(* Logix 5000 AddOnInstructionDefinition export SPEL_Pallet4Get; software revision 30.01 *)

ADD_ON_INSTRUCTION SPEL_ExecCmd   (* revision 1.0 *)
// Executes a command in the robot controller.  Normally this is called by higher level AOIs.
VAR_INPUT
   Start : BOOL; {required}
   MaxTime : DINT := 3000; {required}
END_VAR
VAR_OUTPUT
   InCycle : BOOL; {access Read Only, visible}
   Done : BOOL; {access Read Only, visible}
   Error : BOOL; {access Read Only, visible}
END_VAR
VAR_IN_OUT
   ExtInputs : AB:ETHERNET_MODULE_INT_128Bytes:I:0; {required}
        .DATA[0].0   // ExtCmdGet
        .DATA[0].1   // ExtRespSet
        .DATA[0].2   // ExtCmdResult
        .DATA[0].3   // ExtError
   ExtOutputs : AB:ETHERNET_MODULE_INT_128Bytes:O:0; {required}
        .DATA[0].0   // ExtCmdSet
        .DATA[0].1   // ExtRespGet
        .DATA[0].2   // ExtCmdReset
END_VAR
VAR_INPUT
   Cmd : INT; {required}
   CmdParam1 : INT; {required}
   CmdParam2 : INT; {required}
   CmdParam3 : INT; {required}
   CmdParam4 : INT; {required}
   CmdParam5 : INT; {required}
   CmdParam6 : INT; {required}
   CmdParam7 : INT; {required}
END_VAR
VAR_OUTPUT
   CmdEcho : INT; {access Read Only, visible}
   Resp1 : INT; {access Read Only, visible}
   Resp2 : INT; {access Read Only, visible}
   Resp3 : INT; {access Read Only, visible}
   Resp4 : INT; {access Read Only, visible}
   Resp5 : INT; {access Read Only, visible}
   Resp6 : INT; {access Read Only, visible}
   Resp7 : INT; {access Read Only, visible}
   ErrCode1 : INT; {access Read Only, visible}
   ErrCode2 : INT; {access Read Only, visible}
END_VAR
VAR
   ExtReset : BOOL; {access None}
   ExtError : BOOL; {access None}
   ExtCmdSet : BOOL; {access None}   // Cmd Ready
   ExtCmdGet : BOOL; {access None}   // Cmd Received
   CmdXferDone : BOOL; {access None}
   ExtRespSet : BOOL; {access None}   // Resp Ready
   RespXferDone : BOOL; {access None}
   ExtCmdResult : BOOL; {access None}   // Normal or Error?
   TmrCmdDataRdy : TIMER := (PRE := 5); {access None}
   OneShotDoneOff : BOOL; {access None}
   OneShotStart : BOOL; {access None}
   StartInit : BOOL; {access None}
   OneShotStartError : BOOL; {access None}
   TmrCycle : TIMER := (PRE := 5000); {access None}
   OneshotTmrPreset : BOOL; {access None}
   TmrCmdSet : TIMER := (PRE := 20); {access None}
   OnShotCmdDataXfer : BOOL; {access None}
   OneShotRespDataXfer : BOOL; {access None}
   OneShotDataRdy : BOOL; {access None}
   OtherCmdInCycle : BOOL; {access None}
   s : BOOL; {access None}
   OneShotUnsetCmdIncycle : BOOL; {access None}
   OneShotSetCmdIncycle : BOOL; {access None}
   OneShotSetOtherCmdInCycleError : BOOL; {access None}
   OneShotSetBit : BOOL; {access None}
   MaxTimeError : BOOL; {access None}
END_VAR

ROUTINE Logic   (* ladder *)
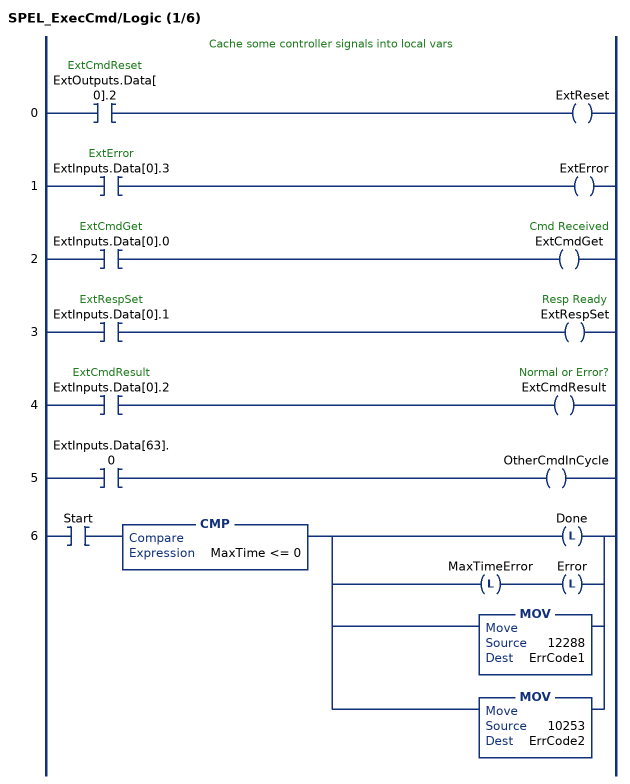
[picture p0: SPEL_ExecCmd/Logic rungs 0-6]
   // Cache some controller signals into local vars
   0: XIC(ExtOutputs.Data[0].2)OTE(ExtReset);
   1: XIC(ExtInputs.Data[0].3)OTE(ExtError);
   2: XIC(ExtInputs.Data[0].0)OTE(ExtCmdGet);
   3: XIC(ExtInputs.Data[0].1)OTE(ExtRespSet);
   4: XIC(ExtInputs.Data[0].2)OTE(ExtCmdResult);
   5: XIC(ExtInputs.Data[63].0)OTE(OtherCmdInCycle);
   6: XIC(Start)CMP(MaxTime <= 0)[OTL(Done) ,OTL(MaxTimeError) OTL(Error) ,MOV(12288,ErrCode1) ,MOV(10253,ErrCode2) ];
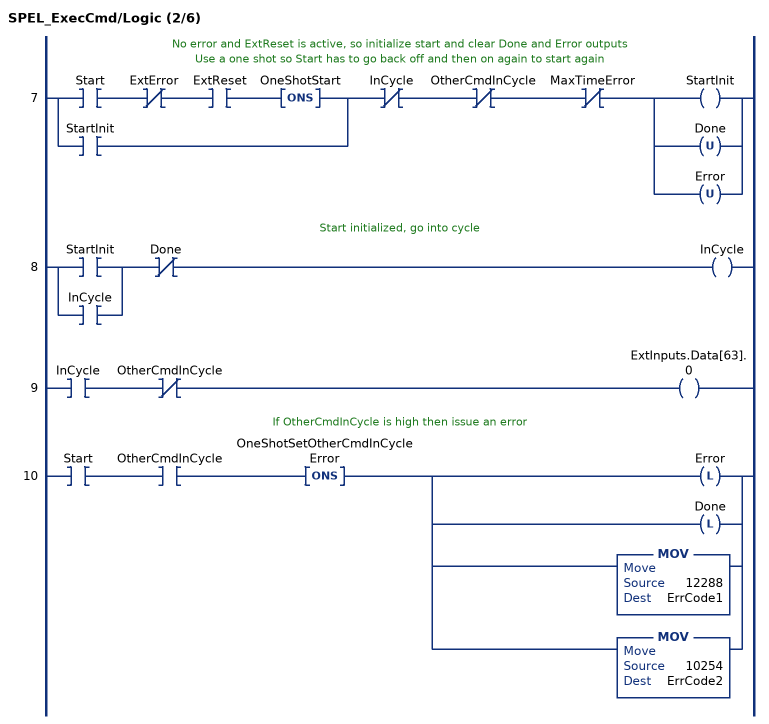
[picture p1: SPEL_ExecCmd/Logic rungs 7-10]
   // No error and ExtReset is active, so initialize start and clear Done and Error outputs
   // Use a one shot so Start has to go back off and then on again to start again
   7: [XIC(Start) XIO(ExtError) XIC(ExtReset) ONS(OneShotStart) ,XIC(StartInit) ]XIO(InCycle)XIO(OtherCmdInCycle)XIO(MaxTimeError)[OTE(StartInit) ,OTU(Done) ,OTU(Error) ];
   // Start initialized, go into cycle
   8: [XIC(StartInit) ,XIC(InCycle) ]XIO(Done)OTE(InCycle);
   9: XIC(InCycle)XIO(OtherCmdInCycle)OTE(ExtInputs.Data[63].0);
   // If OtherCmdInCycle is high then issue an error
   10: XIC(Start)XIC(OtherCmdInCycle)ONS(OneShotSetOtherCmdInCycleError)[OTL(Error) ,OTL(Done) ,MOV(12288,ErrCode1) ,MOV(10254,ErrCode2) ];
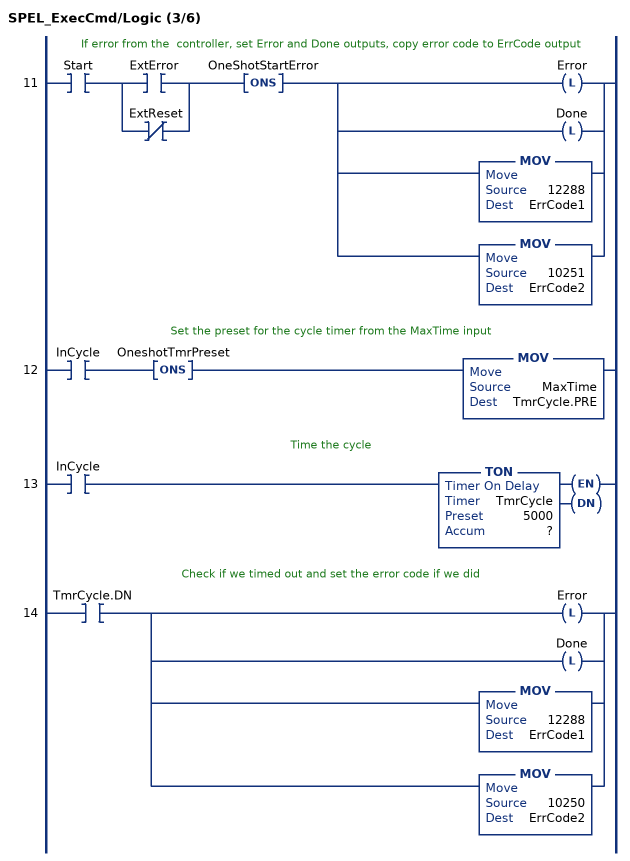
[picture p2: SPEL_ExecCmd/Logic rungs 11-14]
   // If error from the  controller, set Error and Done outputs, copy error code to ErrCode output
   11: XIC(Start)[XIC(ExtError) ,XIO(ExtReset) ]ONS(OneShotStartError)[OTL(Error) ,OTL(Done) ,MOV(12288,ErrCode1) ,MOV(10251,ErrCode2) ];
   // Set the preset for the cycle timer from the MaxTime input
   12: XIC(InCycle)ONS(OneshotTmrPreset)MOV(MaxTime,TmrCycle.PRE);
   // Time the cycle
   13: XIC(InCycle)TON(TmrCycle,?,?);
   // Check if we timed out and set the error code if we did
   14: XIC(TmrCycle.DN)[OTL(Error) ,OTL(Done) ,MOV(12288,ErrCode1) ,MOV(10250,ErrCode2) ];
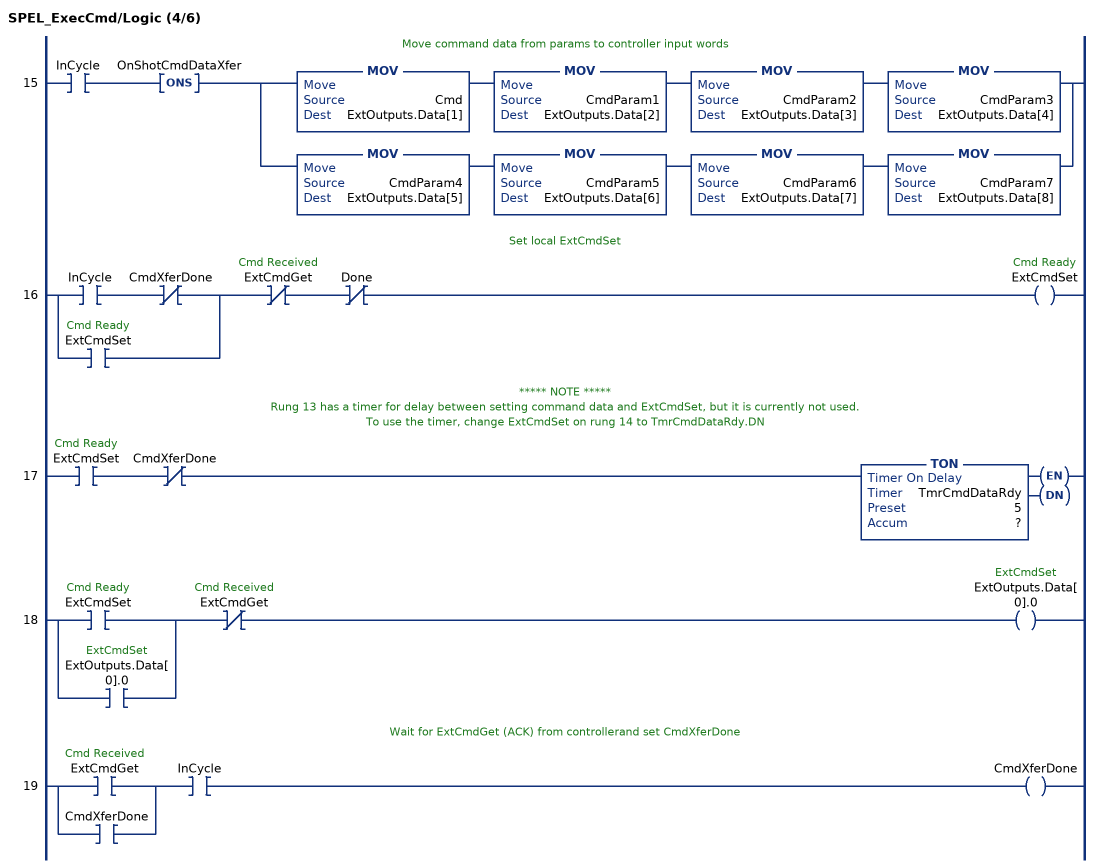
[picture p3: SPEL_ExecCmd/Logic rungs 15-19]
   // Move command data from params to controller input words
   15: XIC(InCycle)ONS(OnShotCmdDataXfer)[MOV(Cmd,ExtOutputs.Data[1]) MOV(CmdParam1,ExtOutputs.Data[2]) MOV(CmdParam2,ExtOutputs.Data[3]) MOV(CmdParam3,ExtOutputs.Data[4]) ,MOV(CmdParam4,ExtOutputs.Data[5]) MOV(CmdParam5,ExtOutputs.Data[6]) MOV(CmdParam6,ExtOutputs.Data[7]) MOV(CmdParam7,ExtOutputs.Data[8]) ];
   // Set local ExtCmdSet
   16: [XIC(InCycle) XIO(CmdXferDone) ,XIC(ExtCmdSet) ]XIO(ExtCmdGet)XIO(Done)OTE(ExtCmdSet);
   // ***** NOTE *****
   // Rung 13 has a timer for delay between setting command data and ExtCmdSet, but it is currently not used.
   // To use the timer, change ExtCmdSet on rung 14 to TmrCmdDataRdy.DN
   17: XIC(ExtCmdSet)XIO(CmdXferDone)TON(TmrCmdDataRdy,?,?);
   18: [XIC(ExtCmdSet) ,XIC(ExtOutputs.Data[0].0) ]XIO(ExtCmdGet)OTE(ExtOutputs.Data[0].0);
   // Wait for ExtCmdGet (ACK) from controllerand set CmdXferDone
   19: [XIC(ExtCmdGet) ,XIC(CmdXferDone) ]XIC(InCycle)OTE(CmdXferDone);
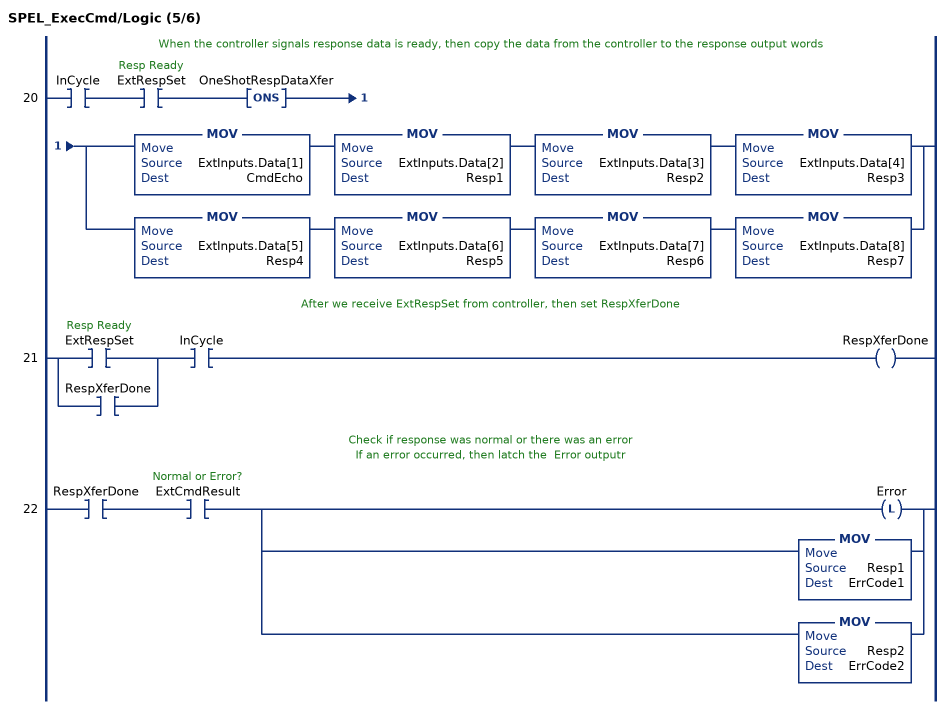
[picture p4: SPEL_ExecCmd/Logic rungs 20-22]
   // When the controller signals response data is ready, then copy the data from the controller to the response output words
   20: XIC(InCycle)XIC(ExtRespSet)ONS(OneShotRespDataXfer)[MOV(ExtInputs.Data[1],CmdEcho) MOV(ExtInputs.Data[2],Resp1) MOV(ExtInputs.Data[3],Resp2) MOV(ExtInputs.Data[4],Resp3) ,MOV(ExtInputs.Data[5],Resp4) MOV(ExtInputs.Data[6],Resp5) MOV(ExtInputs.Data[7],Resp6) MOV(ExtInputs.Data[8],Resp7) ];
   // After we receive ExtRespSet from controller, then set RespXferDone
   21: [XIC(ExtRespSet) ,XIC(RespXferDone) ]XIC(InCycle)OTE(RespXferDone);
   // Check if response was normal or there was an error
   // If an error occurred, then latch the  Error outputr
   22: XIC(RespXferDone)XIC(ExtCmdResult)[OTL(Error) ,MOV(Resp1,ErrCode1) ,MOV(Resp2,ErrCode2) ];
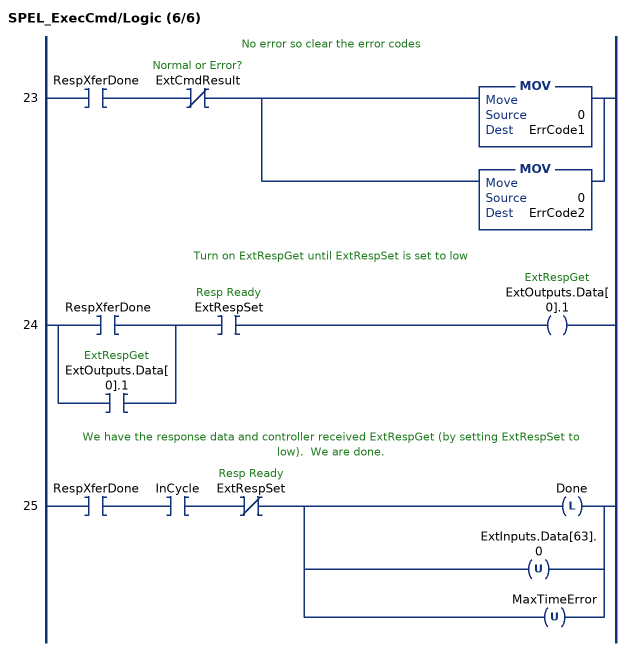
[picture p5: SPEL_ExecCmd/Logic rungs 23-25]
   // No error so clear the error codes
   23: XIC(RespXferDone)XIO(ExtCmdResult)[MOV(0,ErrCode1) ,MOV(0,ErrCode2) ];
   // Turn on ExtRespGet until ExtRespSet is set to low
   24: [XIC(RespXferDone) ,XIC(ExtOutputs.Data[0].1) ]XIC(ExtRespSet)OTE(ExtOutputs.Data[0].1);
   // We have the response data and controller received ExtRespGet (by setting ExtRespSet to low).  We are done.
   25: XIC(RespXferDone)XIC(InCycle)XIO(ExtRespSet)[OTL(Done) ,OTU(ExtInputs.Data[63].0) ,OTU(MaxTimeError) ];
END_ROUTINE
END_ADD_ON_INSTRUCTION

ADD_ON_INSTRUCTION SPEL_Pallet4Get   (* revision 1.2, vendor SEIKO EPSON CORP. *)
// Acquires the details of 4-point definition of the specified pallet.
VAR_OUTPUT
   InCycle : BOOL; {access None, visible}
   Done : BOOL; {access None, visible}
   Error : BOOL; {access None, visible}
END_VAR
VAR_INPUT
   Start : BOOL; {access None, required}
   PalletNum : INT; {access None, required}
   Point1 : INT; {access Read Only, required}
   Point2 : INT; {access None, required}
   Point3 : INT; {access None, required}
   Point4 : INT; {access Read Only, required}
END_VAR
VAR_OUTPUT
   Rows : INT; {access Read Only, visible}
   Columns : INT; {access Read Only, visible}
END_VAR
VAR_IN_OUT
   ExtInputs : AB:ETHERNET_MODULE_INT_128Bytes:I:0; {required}
   ExtOutputs : AB:ETHERNET_MODULE_INT_128Bytes:O:0; {required}
END_VAR
VAR_OUTPUT
   ErrCode1 : INT; {access None, visible}
   ErrCode2 : INT; {access None, visible}
END_VAR
VAR
   ExecGetPallet : SPEL_ExecCmd := (MaxTime := 3000); {access None}
   ExecTimeout : DINT; {access None}
   CmdParam2 : INT; {access None}
   CmdParam3 : INT; {access None}
   CmdParam4 : INT; {access None}
   CmdParam5 : INT; {access None}
   CmdParam6 : INT; {access None}
   CmdParam7 : INT; {access None}
END_VAR

ROUTINE Logic   (* ladder *)
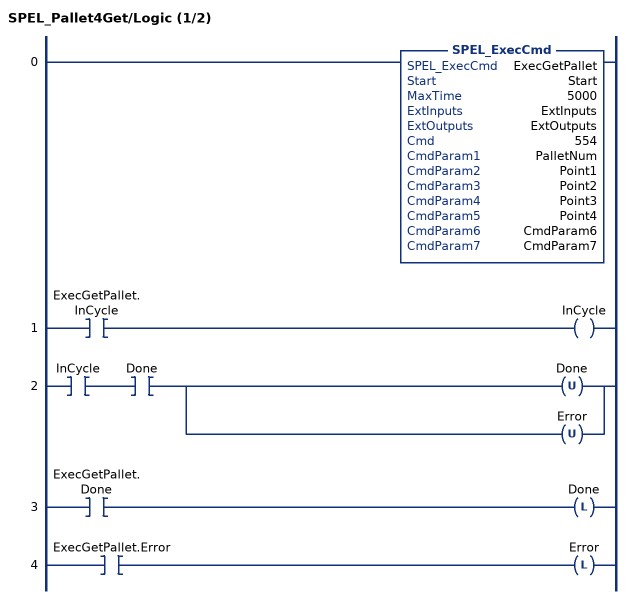
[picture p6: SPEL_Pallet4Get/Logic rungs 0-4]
   0: SPEL_ExecCmd(ExecGetPallet,Start,5000,ExtInputs,ExtOutputs,554,PalletNum,Point1,Point2,Point3,Point4,CmdParam6,CmdParam7);
   1: XIC(ExecGetPallet.InCycle)OTE(InCycle);
   2: XIC(InCycle)XIC(Done)[OTU(Done) ,OTU(Error) ];
   3: XIC(ExecGetPallet.Done)OTL(Done);
   4: XIC(ExecGetPallet.Error)OTL(Error);
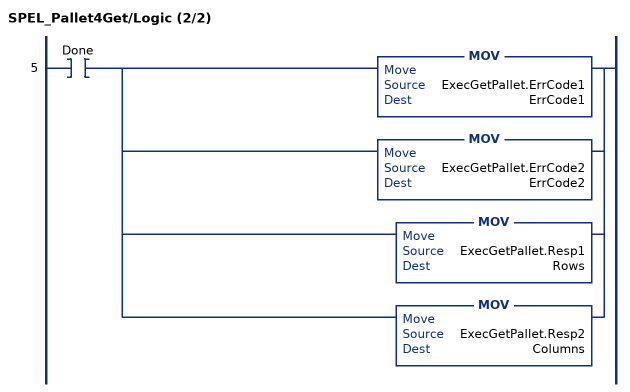
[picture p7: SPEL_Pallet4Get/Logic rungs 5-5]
   5: XIC(Done)[MOV(ExecGetPallet.ErrCode1,ErrCode1) ,MOV(ExecGetPallet.ErrCode2,ErrCode2) ,MOV(ExecGetPallet.Resp1,Rows) ,MOV(ExecGetPallet.Resp2,Columns) ];
END_ROUTINE
END_ADD_ON_INSTRUCTION
